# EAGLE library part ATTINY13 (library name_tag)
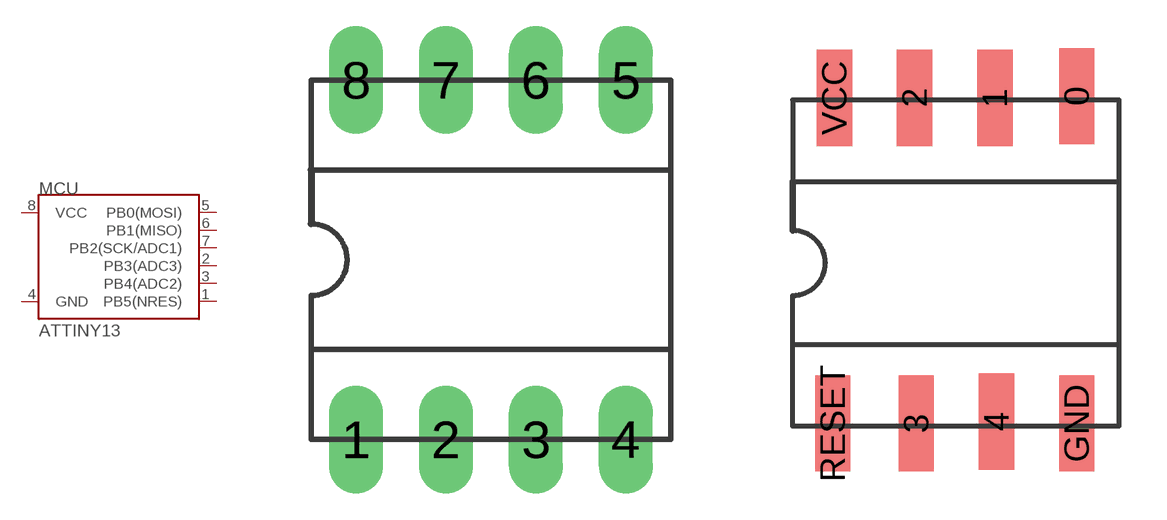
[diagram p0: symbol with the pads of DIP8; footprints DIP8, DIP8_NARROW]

Designator prefix MCU

## ATTINY13  [DIP8]
1  PB5(NRES)
2  PB3(ADC3)
3  PB4(ADC2)
4  GND
5  PB0(MOSI)
6  PB1(MISO)
7  PB2(SCK/ADC1)
8  VCC

## ATTINY13DIP8_NARROW  [DIP8_NARROW]
0  PB0(MOSI)
1  PB1(MISO)
2  PB2(SCK/ADC1)
3  PB3(ADC3)
4  PB4(ADC2)
GND  GND
RESET  PB5(NRES)
VCC  VCC

## Footprint DIP8 (pad centres in mm)
drill 1.016 long: 1 -5.08,-5.08; 2 -2.54,-5.08; 3 0,-5.08; 4 2.54,-5.08; 5 2.54,5.08; 6 0,5.08; 7 -2.54,5.08; 8 -5.08,5.08

## Footprint DIP8_NARROW (pad centres in mm)
smd 1.1 x 3: 0 5.8,5.8; 1 3.25,5.75; 2 0.75,5.75; 3 0.8,-4.4; 4 3.3,-4.35; GND 5.8,-4.4; RESET -1.8,-4.4; VCC -1.75,5.75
